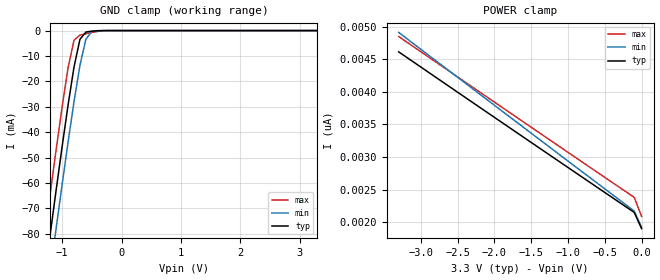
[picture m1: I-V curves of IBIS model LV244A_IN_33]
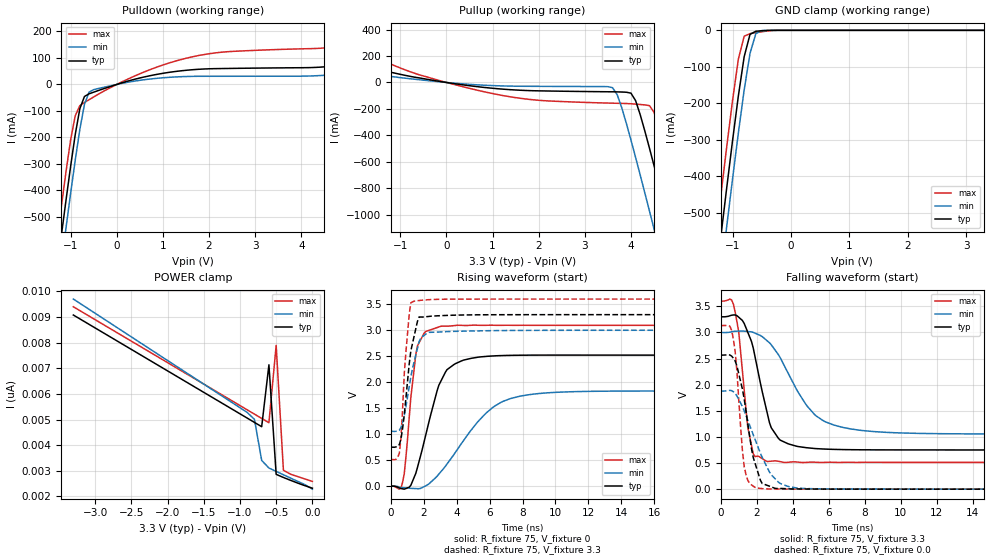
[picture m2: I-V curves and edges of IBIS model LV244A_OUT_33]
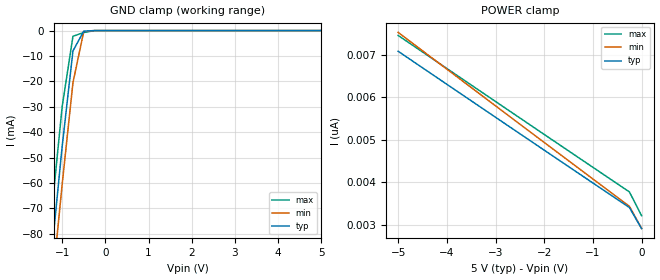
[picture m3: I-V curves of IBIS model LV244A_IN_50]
| TEXAS INSTRUMENTS INCORPORATED
| Standard Linear and Logic Group
| IBIS Model of SN74LV244A
| OCTAL BUFFER/DRIVER WITH 3-STATE OUTPUTS
| SOIC 20-pin (DW), SOP 20-pin (NS), SSOP 20-pin (DB), TSSOP 20-pin (PW)
| and TVSOP 20-pin (DGV) Package
[IBIS Ver]   3.2
[Comment Char]  |_char
[File Name]   lv244a.ibs
[File Rev]   2.0 I_die
[Date]   May 31, 2001
[Source]   Data created from HSPICE simulations at TI-SLL.
[Notes]   The following is an IBIS list for the LV244A.
|   Please contact sllibis@ti.com with questions and
|   comments concerning SLL IBIS models.
|   The warning about non-monotonic V-I curves might be reported,
|   but it is nano ampere region and negligible.
|   The warning about AC Rising Endpoint might be reported,
|   but it is due to HSPICE issue and negligible.
[Disclaimer] Property of Texas Instruments Incorporated.  Unauthorized
   reproduction and/or distribution is strictly prohibited.
   This product is protected under copyright law.
   Created 2001, (C) Copyright 2001, Texas Instruments Inc.,
   All Rights Reserved.
   UNLESS THERE IS A SIGNED, WRITTEN AGREEMENT TO THE
   CONTRARY, TEXAS INSTRUMENTS ("TI") IS PROVIDING THE IBIS
   MODELS "AS IS" AND WITHOUT ANY WARRANTY, EXPRESSED OR
   IMPLIED.  TI assumes no liability for:
   1) the accuracy of the IBIS models provided to your
   company;
   2) the proper functioning of these IBIS Models in your
   design or for any resulting applications; or
   3) infringement of patents, copyrights or intellectual
   property rights resulting from your use of these IBIS
   models.
   TI provides IBIS Models as a service to our customers.
   You and your company shall not distribute, sell or give
   these models to anyone else without prior written
   permission from TI.
   TI reserves the right to make changes to our products or
   to discontinue any semiconductor product or service
   without notice, and advises our customers to obtain the
   latest version of relevant information to verify, before
   placing orders, that the information being relied on is
   current.
   Please be aware that your receipt and use of the IBIS
   information provided shall serve as acceptance of these
   terms and conditions.  If you do not accept these terms,
   you should return or destroy the IBIS models and any
   other accompanying information immediately.
|   Component LV244A_DW
[Component]   LV244A_DW
[Manufacturer]  Texas Instruments, Inc.
[Package]
|   typ   min   max
R_pkg   0.038   0.033   0.045
L_pkg   5.012nH   4.110nH   6.349nH
C_pkg   0.717pF   0.530pF   0.868pF
[Pin]   signal_name   model_name   R_pin   L_pin   C_pin
1   1OE_NOT   LV244A_IN   0.042   6.336nH   0.865pF
2   1A1   LV244A_IN   0.043   5.542nH   0.867pF
3   2Y4   LV244A_OUT   0.034   4.714nH   0.732pF
4   1A2   LV244A_IN   0.034   4.377nH   0.591pF
5   2Y3   LV244A_OUT   0.036   4.130nH   0.533pF
6   1A3   LV244A_IN   0.035   4.111nH   0.530pF
7   2Y2   LV244A_OUT   0.034   4.284nH   0.583pF
8   1A4   LV244A_IN   0.034   4.634nH   0.726pF
9   2Y1   LV244A_OUT   0.040   5.518nH   0.865pF
10   GND   GND   0.043   6.349nH   0.866pF
11   2A1   LV244A_IN   0.041   6.281nH   0.861pF
12   1Y4   LV244A_OUT   0.045   5.561nH   0.868pF
13   2A2   LV244A_IN   0.033   4.778nH   0.742pF
14   1Y3   LV244A_OUT   0.035   4.414nH   0.596pF
15   2A3   LV244A_IN   0.035   4.110nH   0.533pF
16   1Y2   LV244A_OUT   0.036   4.130nH   0.533pF
17   2A4   LV244A_IN   0.034   4.377nH   0.591pF
18   1Y1   LV244A_OUT   0.034   4.714nH   0.731pF
19   2OE_NOT   LV244A_IN   0.043   5.569nH   0.868pF
20   VCC   POWER   0.042   6.308nH   0.864pF
|   Component LV244A_NS
[Component]   LV244A_NS
[Manufacturer]  Texas Instruments, Inc.
[Package]
|   typ   min   max
R_pkg   0.044   0.029   0.058
L_pkg   3.666nH   2.317nH   5.115nH
C_pkg   0.548pF   0.316pF   0.725pF
[Pin]   signal_name   model_name   R_pin   L_pin   C_pin
1   1OE_NOT   LV244A_IN   0.058   5.115nH   0.725pF
2   1A1   LV244A_IN   0.053   4.591nH   0.724pF
3   2Y4   LV244A_OUT   0.049   3.754nH   0.572pF
4   1A2   LV244A_IN   0.029   2.549nH   0.388pF
5   2Y3   LV244A_OUT   0.031   2.317nH   0.316pF
6   1A3   LV244A_IN   0.031   2.317nH   0.316pF
7   2Y2   LV244A_OUT   0.029   2.556nH   0.399pF
8   1A4   LV244A_IN   0.049   3.754nH   0.579pF
9   2Y1   LV244A_OUT   0.053   4.591nH   0.724pF
10   GND   GND   0.058   5.115nH   0.725pF
11   2A1   LV244A_IN   0.058   5.115nH   0.725pF
12   1Y4   LV244A_OUT   0.053   4.591nH   0.724pF
13   2A2   LV244A_IN   0.049   3.754nH   0.579pF
14   1Y3   LV244A_OUT   0.029   2.557nH   0.399pF
15   2A3   LV244A_IN   0.031   2.317nH   0.316pF
16   1Y2   LV244A_OUT   0.031   2.317nH   0.316pF
17   2A4   LV244A_IN   0.029   2.557nH   0.399pF
18   1Y1   LV244A_OUT   0.049   3.754nH   0.579pF
19   2OE_NOT   LV244A_IN   0.053   4.591nH   0.724pF
20   VCC   POWER   0.058   5.115nH   0.725pF
|   Component LV244A_DB
[Component]   LV244A_DB
[Manufacturer]  Texas Instruments, Inc.
[Package]
|   typ   min   max
R_pkg   0.040   0.035   0.051
L_pkg   3.495nH   3.035nH   4.314nH
C_pkg   0.420pF   0.346pF   0.502pF
[Pin]   signal_name   model_name   R_pin   L_pin   C_pin
1   1OE_NOT   LV244A_IN   0.049   4.310nH   0.502pF
2   1A1   LV244A_IN   0.048   3.903nH   0.487pF
3   2Y4   LV244A_OUT   0.035   3.189nH   0.396pF
4   1A2   LV244A_IN   0.035   3.036nH   0.347pF
5   2Y3   LV244A_OUT   0.035   3.035nH   0.367pF
6   1A3   LV244A_IN   0.035   3.035nH   0.367pF
7   2Y2   LV244A_OUT   0.035   3.036nH   0.347pF
8   1A4   LV244A_IN   0.035   3.189nH   0.397pF
9   2Y1   LV244A_OUT   0.047   3.899nH   0.488pF
10   GND   GND   0.051   4.314nH   0.500pF
11   2A1   LV244A_IN   0.051   4.314nH   0.500pF
12   1Y4   LV244A_OUT   0.047   3.899nH   0.488pF
13   2A2   LV244A_IN   0.035   3.189nH   0.397pF
14   1Y3   LV244A_OUT   0.035   3.036nH   0.346pF
15   2A3   LV244A_IN   0.035   3.035nH   0.367pF
16   1Y2   LV244A_OUT   0.035   3.035nH   0.367pF
17   2A4   LV244A_IN   0.035   3.036nH   0.346pF
18   1Y1   LV244A_OUT   0.035   3.189nH   0.397pF
19   2OE_NOT   LV244A_IN   0.047   3.899nH   0.488pF
20   VCC   POWER   0.051   4.314nH   0.502pF
|   Component LV244A_PW
[Component]   LV244A_PW
[Manufacturer]  Texas Instruments, Inc.
[Package]
|   typ   min   max
R_pkg   0.035   0.024   0.047
L_pkg   2.399nH   1.710nH   3.250nH
C_pkg   0.284pF   0.166pF   0.418pF
[Pin]   signal_name   model_name   R_pin   L_pin   C_pin
1   1OE_NOT   LV244A_IN   0.041   3.102nH   0.410pF
2   1A1   LV244A_IN   0.040   2.777nH   0.363pF
3   2Y4   LV244A_OUT   0.029   2.194nH   0.260pF
4   1A2   LV244A_IN   0.025   1.710nH   0.166pF
5   2Y3   LV244A_OUT   0.025   1.740nH   0.191pF
6   1A3   LV244A_IN   0.024   1.763nH   0.193pF
7   2Y2   LV244A_OUT   0.024   1.817nH   0.174pF
8   1A4   LV244A_IN   0.028   2.256nH   0.265pF
9   2Y1   LV244A_OUT   0.045   2.887nH   0.368pF
10   GND   GND   0.047   3.250nH   0.417pF
11   2A1   LV244A_IN   0.046   3.244nH   0.418pF
12   1Y4   LV244A_OUT   0.046   2.961nH   0.375pF
13   2A2   LV244A_IN   0.033   2.334nH   0.268pF
14   1Y3   LV244A_OUT   0.029   1.915nH   0.179pF
15   2A3   LV244A_IN   0.031   1.934nH   0.203pF
16   1Y2   LV244A_OUT   0.032   1.917nH   0.201pF
17   2A4   LV244A_IN   0.030   1.833nH   0.173pF
18   1Y1   LV244A_OUT   0.036   2.324nH   0.268pF
19   2OE_NOT   LV244A_IN   0.042   2.869nH   0.372pF
20   VCC   POWER   0.042   3.160nH   0.414pF
|   Component LV244A_DGV
[Component]   LV244A_DGV
[Manufacturer]  Texas Instruments, Inc.
[Package]
|   typ   min   max
R_pkg   0.044   0.038   0.048
L_pkg   2.561nH   2.236nH   2.961nH
C_pkg   0.342pF   0.264pF   0.446pF
[Pin]   signal_name   model_name   R_pin   L_pin   C_pin
1   1OE_NOT   LV244A_IN   0.044   2.935nH   0.417pF
2   1A1   LV244A_IN   0.042   2.869nH   0.446pF
3   2Y4   LV244A_OUT   0.043   2.399nH   0.316pF
4   1A2   LV244A_IN   0.044   2.236nH   0.265pF
5   2Y3   LV244A_OUT   0.046   2.278nH   0.264pF
6   1A3   LV244A_IN   0.045   2.274nH   0.264pF
7   2Y2   LV244A_OUT   0.044   2.285nH   0.269pF
8   1A4   LV244A_IN   0.043   2.452nH   0.320pF
9   2Y1   LV244A_OUT   0.044   2.900nH   0.446pF
10   GND   GND   0.044   2.961nH   0.418pF
11   2A1   LV244A_IN   0.045   2.954nH   0.418pF
12   1Y4   LV244A_OUT   0.042   2.847nH   0.443pF
13   2A2   LV244A_IN   0.045   2.453nH   0.319pF
14   1Y3   LV244A_OUT   0.045   2.297nH   0.269pF
15   2A3   LV244A_IN   0.048   2.334nH   0.268pF
16   1Y2   LV244A_OUT   0.048   2.335nH   0.267pF
17   2A4   LV244A_IN   0.046   2.299nH   0.268pF
18   1Y1   LV244A_OUT   0.046   2.457nH   0.320pF
19   2OE_NOT   LV244A_IN   0.043   2.848nH   0.441pF
20   VCC   POWER   0.038   2.812nH   0.408pF
[Model Selector]   LV244A_IN
LV244A_IN_33   3.3-V Vcc Input Model
LV244A_IN_50   5.0-V Vcc Input Model
[Model Selector]   LV244A_OUT
LV244A_OUT_33   3.3-V Vcc Output Model
LV244A_OUT_50   5.0-V Vcc Output Model
| Models and submodels in the file (4): LV244A_IN_33 (Input), LV244A_OUT_33 (3-state), LV244A_IN_50 (Input), LV244A_OUT_50 (3-state)
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|   Model LV244A_IN_33
[Model]   LV244A_IN_33
Model_type  Input
Polarity   Inverting
Vinl = 0.99
Vinh = 2.31
| variable   typ   min   max
C_comp   1.33pf   1.00pf   1.66pf
[Temperature Range]   25   85   -40
[Voltage Range]   3.3   3.0   3.6
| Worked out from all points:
|   GND clamp passes 1 mA (typ) near -0.61 V on its own axis
[GND Clamp]
|   Voltage   I(typ)   I(min)   I(max)
-3.3V     -460.4mA   -474.6mA   -445.4mA
-1.3V     -97.49mA   -112.5mA   -81.51mA
-1.2V     -79.93mA   -94.98mA   -63.94mA
-1.1V     -62.59mA   -77.62mA   -46.67mA
-1V       -45.6mA    -60.54mA   -29.97mA
-900mV    -29.25mA   -43.87mA   -14.58mA
-800mV    -14.28mA   -27.95mA   -3.811mA
-700mV    -3.418mA   -13.61mA   -1.784mA
-600mV    -581.1uA   -3.398mA   -1.247mA
-500mV    -232.6uA   -352.5uA   -758.6uA
-400mV    -58.12uA   -21.94uA   -324.1uA
3.3V      1.902nA    2.343nA    1.692nA
[POWER Clamp]
|   Voltage   I(typ)   I(min)   I(max)
-3.3V     4.612nA    4.91nA     4.847nA
-1.6V     3.301nA    3.451nA    3.534nA
-100mV    2.151nA    2.173nA    2.382nA
0V        1.902nA    1.921nA    2.089nA
|   Model LV244A_OUT_33
[Model]   LV244A_OUT_33
Model_type  3-state
Polarity   Non-Inverting
Enable   Active-Low
Vmeas = 1.65v
Cref = 15pf
| variable   typ   min   max
C_comp   5.80pf   4.35pf   7.25pf
[Temperature Range]   25   85   -40
[Voltage Range]   3.3   3.0   3.6
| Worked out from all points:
|   slope of the pulldown table from 0 to 0.495 V, typ, clamps not added: 20.5 ohm
|   slope of the pullup table from 0 to 0.495 V, typ, clamps not added: 20.4 ohm
|   GND clamp passes 1 mA (typ) near -0.48 V on its own axis
|   rising waveform, R_fixture 75, V_fixture 0: 20-80 % time 1.3ns typ, 2.74ns min, 564ps max; typ from 0 V to 2.52 V
|   falling waveform, R_fixture 75, V_fixture 3.3: 20-80 % time 984ps typ, 2.05ns min, 525ps max; typ from 3.3 V to 0.75 V
|   rising waveform, R_fixture 75, V_fixture 3.3: 20-80 % time 576ps typ, 721ps min, 376ps max; typ from 0.75 V to 3.3 V
|   falling waveform, R_fixture 75, V_fixture 0.0: 20-80 % time 782ps typ, 1.34ns min, 406ps max; typ from 2.57 V to 0 V
[Pulldown]
|   Voltage   I(typ)   I(min)   I(max)
-3.3V     -3.499A    -3.598A    -3.395A
-1.3V     -703.2mA   -808.1mA   -592.6mA
-1.2V     -568.8mA   -673.6mA   -458.9mA
-1.1V     -436.7mA   -540.9mA   -329.1mA
-900mV    -189mA     -285.6mA   -118.2mA
-800mV    -91.12mA   -169.3mA   -79.79mA
-700mV    -45.31mA   -74.84mA   -67.84mA
-600mV    -35.38mA   -28.89mA   -57.56mA
-500mV    -29.09mA   -19.5mA    -47.13mA
1.7V      56.34mA    30.69mA    106.6mA
4.6V      67.98mA    35.58mA    139.6mA
6.6V      107.3mA    55.93mA    212.1mA
[Pullup]
|   Voltage   I(typ)   I(min)   I(max)
-3.3V     218mA      119.5mA    409.1mA
600mV     -28.8mA    -16.43mA   -52.81mA
3.6V      -70.47mA   -39.38mA   -156.4mA
3.8V      -72.1mA    -190.8mA   -158mA
4V        -80.77mA   -435.4mA   -160.7mA
4.1V      -137.2mA   -566mA     -163.4mA
4.4V      -495.5mA   -969.8mA   -174.7mA
4.5V      -628.3mA   -1.107A    -225.3mA
4.8V      -1.037A    -1.521A    -593.5mA
5.1V      -1.452A    -1.939A    -1.003A
5.2V      -1.592A    -2.079A    -1.141A
6.6V      -3.561A    -4.049A    -3.11A
[GND Clamp]
|   Voltage   I(typ)   I(min)   I(max)
-3.3V     -3.499A    -3.598A    -3.395A
-1.3V     -700.7mA   -806.6mA   -588.2mA
-1.2V     -565.8mA   -671.8mA   -453.1mA
-1.1V     -432.8mA   -538.7mA   -320.5mA
-1V       -303.2mA   -408.1mA   -193.1mA
-900mV    -179.9mA   -281.7mA   -79.14mA
-800mV    -72.03mA   -163.1mA   -16.09mA
-700mV    -10.91mA   -62.8mA    -9.073mA
-600mV    -2.488mA   -8.975mA   -6.418mA
-500mV    -1.18mA    -669.4uA   -3.989mA
-200mV    -3.043nA   -62.36nA   -8.636uA
3.3V      2.32nA     2.714nA    2.306nA
[POWER Clamp]
|   Voltage   I(typ)   I(min)   I(max)
-3.3V     9.075nA    9.698nA    9.397nA
-900mV    5.055nA    5.276nA    5.377nA
-800mV    4.888nA    5.006nA    5.21nA
-700mV    4.719nA    3.405nA    5.043nA
-600mV    7.133nA    3.107nA    4.875nA
-500mV    2.861nA    2.976nA    7.89nA
-400mV    2.739nA    2.845nA    3.022nA
-300mV    2.626nA    2.714nA    2.864nA
-100mV    2.416nA    2.455nA    2.678nA
0V        2.32nA     2.283nA    2.585nA
[Ramp]
| variable   typ   min   max
dV/dt_r  1.5173E+00/1.2644E-09  1.1094E+00/2.7725E-09  1.8598E+00/5.6834E-10
dV/dt_f  1.5520E+00/9.7287E-10  1.1828E+00/2.0465E-09  1.8771E+00/5.5709E-10
R_load = 75
[Rising Waveform]
R_fixture = 75
V_fixture = 0
|   Time   V(typ)   V(min)   V(max)
0s        0V         0V         0V
700ps     -50.74mV   -27.92mV   77.76mV
1.5ns     245.6mV    -45.81mV   2.523V
2.1ns     975.2mV    6.901mV    2.975V
2.9ns     1.939V     230.4mV    3.063V
3.3ns     2.191V     383mV      3.08V
4.8ns     2.455V     1.051V     3.095V
6.3ns     2.508V     1.541V     3.096V
8.5ns     2.521V     1.765V     3.095V
25ns      2.521V     1.831V     3.094V
[Falling Waveform]
R_fixture = 75
V_fixture = 3.3
V_fixture_min = 3.0
V_fixture_max = 3.6
|   Time   V(typ)   V(min)   V(max)
0s        3.3V       3V         3.6V
700ps     3.334V     3.018V     3.539V
1ns       3.289V     3.025V     2.993V
1.5ns     3V         3.017V     1.176V
1.8ns     2.703V     3.001V     678.5mV
2.5ns     1.571V     2.86V      540.2mV
3.3ns     938.2mV    2.515V     526.5mV
5.2ns     778.5mV    1.431V     516.4mV
6.7ns     758.1mV    1.188V     512.4mV
25ns      750mV      1.055V     512.3mV
[Rising Waveform]
R_fixture = 75
V_fixture = 3.3
V_fixture_min = 3.0
V_fixture_max = 3.6
|   Time   V(typ)   V(min)   V(max)
0s        750mV      1.055V     512.3mV
500ps     802mV      1.075V     631.5mV
600ps     904.1mV    1.132V     926mV
800ps     1.371V     1.361V     2.158V
1.1ns     2.346V     1.91V      3.299V
1.2ns     2.603V     2.103V     3.528V
1.4ns     2.885V     2.392V     3.56V
1.7ns     3.255V     2.775V     3.572V
2.3ns     3.266V     2.96V      3.589V
25ns      3.3V       3V         3.6V
[Falling Waveform]
R_fixture = 75
V_fixture = 0.0
|   Time   V(typ)   V(min)   V(max)
0s        2.566V     1.878V     3.131V
600ps     2.546V     1.885V     3.039V
800ps     2.45V      1.832V     2.62V
1.3ns     1.723V     1.499V     430mV
1.7ns     780.1mV    1.133V     81.67mV
2ns       387.8mV    864.4mV    22.01mV
2.3ns     107.3mV    606.7mV    10.73mV
2.8ns     43.83mV    276.7mV    4.371mV
4.3ns     4.652mV    20.03mV    1.256mV
25ns      25.98uV    16.44uV    15.85uV
|   Model LV244A_IN_50
[Model]   LV244A_IN_50
Model_type  Input
Polarity   Inverting
Vinl = 1.5
Vinh = 3.5
| variable   typ   min   max
C_comp   1.33pf   1.00pf   1.66pf
[Temperature Range]   25   85   -40
[Voltage Range]   5.0   4.5   5.5
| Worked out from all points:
|   GND clamp passes 1 mA (typ) near -0.52 V on its own axis
[GND Clamp]
|   Voltage   I(typ)   I(min)   I(max)
-5V       -772.7mA   -786.5mA   -758.1mA
-1.5V     -133mA     -148mA     -117.2mA
-1.25V    -88.68mA   -103.7mA   -72.7mA
-1V       -45.6mA    -60.54mA   -29.97mA
-750mV    -7.993mA   -20.49mA   -2.232mA
-500mV    -232.6uA   -352.5uA   -758.6uA
-250mV    -2.633nA   -182.1nA   -26.9uA
5V        2.904nA    3.644nA    2.541nA
[POWER Clamp]
|   Voltage   I(typ)   I(min)   I(max)
-5V       7.079nA    7.524nA    7.451nA
-2.5V     5.139nA    5.363nA    5.509nA
-250mV    3.401nA    3.43nA     3.769nA
0V        2.904nA    2.91nA     3.209nA
